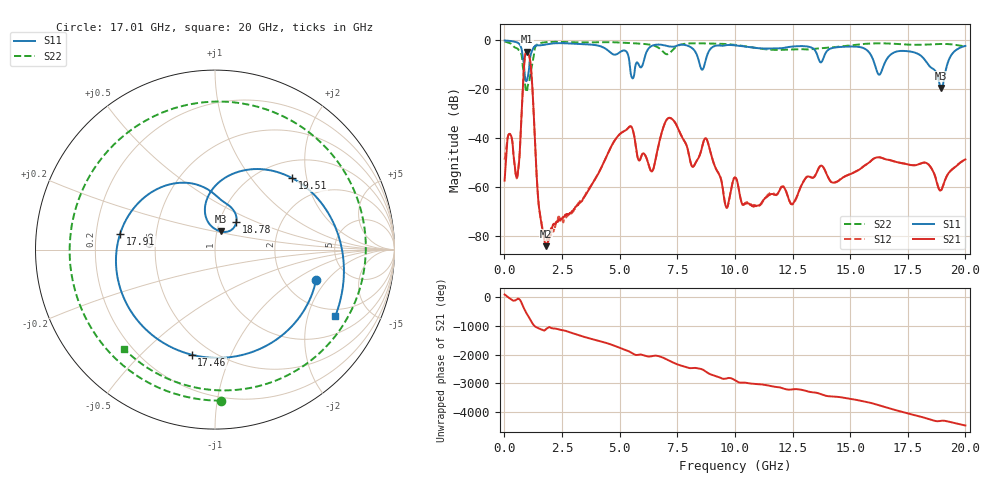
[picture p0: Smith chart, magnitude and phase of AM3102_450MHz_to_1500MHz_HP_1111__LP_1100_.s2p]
!Agilent Technologies,E8364B,MY43040894,A.07.50.67
!Agilent E8364B: A.07.50.67
!Date: Thursday, January 11, 2018 06:51:57
!Correction: S11(Full 2 Port(1,2))
!S21(Full 2 Port(1,2))
!S12(Full 2 Port(1,2))
!S22(Full 2 Port(1,2))
!S2P File: Measurements: S11, S21, S12, S22:
# Hz S  dB  R 50
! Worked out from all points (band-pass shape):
!   1601 points, 10 MHz to 20 GHz, reference 50 ohm
!   highest |S21| = -4.68 dB at 972 MHz (marker M1); lowest = -84.4 dB at 1.809 GHz (marker M2)
!   |S21| within 3 dB of the highest: 879.9 MHz to 1.106 GHz (226 MHz wide, 22.8 % of centre)
!   lowest |S11| = -19.5 dB at 18.95 GHz (marker M3), VSWR 1.24, Z = 52.1 + j10.7 ohm
!   |S11| at or under -10 dB: 5.436 GHz to 5.695 GHz (258.2 MHz wide, 4.64 % of centre); 16.07 GHz to 16.47 GHz (397.1 MHz wide, 2.44 % of centre); 18.39 GHz to 19.21 GHz (817.8 MHz wide, 4.35 % of centre)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
!   |S22| runs from -21.3 to -0.5 dB; largest |S21 - S12| = 0.0023
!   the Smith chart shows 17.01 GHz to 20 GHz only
!   S11 on the Smith chart (normalised r, x): 17.01 GHz: 3.00, -1.53; 17.46 GHz: 0.40, -0.72; 17.91 GHz: 0.30, +0.08; 18.78 GHz: 1.20, +0.39; 19.51 GHz: 1.36, +1.65; 20 GHz: 1.68, -3.02
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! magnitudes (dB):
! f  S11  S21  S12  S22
! 10 MHz  -0.1  -57.5  -48.9  -0.5
! 234.9 MHz  -0.3  -38.4  -38.3  -1.1
! 572.2 MHz  -1.0  -55.2  -55.5  -3.4
! 972 MHz  -16.5  -4.7  -4.7  -21.2
! 1.522 GHz  -2.1  -69.7  -69.8  -1.2
! 1.809 GHz  -1.7  -84.4  -81.8  -0.8
! 3.346 GHz  -1.6  -66.0  -65.4  -0.9
! 5.395 GHz  -7.1  -35.6  -35.6  -1.1
! 6.682 GHz  -1.7  -43.2  -43.2  -3.0
! 7.219 GHz  -2.6  -31.9  -31.9  -4.8
! 8.781 GHz  -6.5  -40.6  -40.7  -1.3
! 9.63 GHz  -2.0  -68.4  -68.6  -1.5
! 10.01 GHz  -2.1  -56.2  -56.2  -1.9
! 13.34 GHz  -3.1  -56.4  -56.2  -3.6
! 16.68 GHz  -6.6  -49.0  -49.0  -1.3
! 17.01 GHz  -4.6  -49.9  -49.9  -1.5
! 17.46 GHz  -4.4  -50.8  -50.8  -1.7
! 17.91 GHz  -5.4  -51.0  -50.9  -1.8
! 18.78 GHz  -14.2  -58.8  -58.6  -1.6
! 18.95 GHz  -19.5  -61.3  -61.5  -1.5
! 19.51 GHz  -4.6  -52.3  -52.1  -1.8
! 20 GHz  -2.3  -48.8  -48.9  -2.5
